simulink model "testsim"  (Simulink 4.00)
settings: Solver=ode23  StartTime=0.0  StopTime=600  MaxStep=.1  RelTol=1e-3
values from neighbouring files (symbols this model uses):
  c1 = 3    [scensim.m]
  l1 = 3    [scensim.m]
  v1 = 0.92    [scensim.m]
undefined symbols (not defined in the file or in its folder): c0, l0, p, tcap, tload, tvref, v0, x0

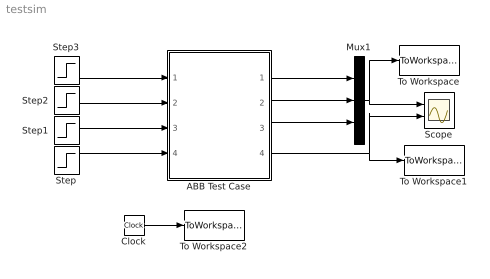
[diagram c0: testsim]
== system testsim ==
  ABB Test Case : Subsystem
  Clock : Clock
  Mux1 : Mux  Inputs=3
  Scope : Scope  NumInputPorts=2
  Step : Step  Time=100  Before=0  After=1  SampleTime=0
  Step1 : Step  Time=tvref  Before=v0  After=v1  SampleTime=0
  Step2 : Step  Time=tload  Before=l0  After=l1  SampleTime=0
  Step3 : Step  Time=tcap  Before=c0  After=c1  SampleTime=0
  To Workspace : ToWorkspace  VariableName=V  SampleTime=-1  SaveFormat=Array
  To Workspace1 : ToWorkspace  VariableName=Efd  SampleTime=-1  SaveFormat=Array
  To Workspace2 : ToWorkspace  VariableName=t  SampleTime=-1  SaveFormat=Array
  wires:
  Step2/1 -> ABB Test Case/2(LoadStep)
  Step3/1 -> ABB Test Case/1(CapStep)
  Step1/1 -> ABB Test Case/3(TapVref)
  Step/1 -> ABB Test Case/4(faulted)
  ABB Test Case/1(V2) -> Mux1/1
  ABB Test Case/2(V3) -> Mux1/2
  ABB Test Case/3(V4) -> Mux1/3
  Mux1/1 -> Scope/1, To Workspace/1
  Clock/1 -> To Workspace2/1
  ABB Test Case/4(G1Efd) -> To Workspace1/1, Scope/2

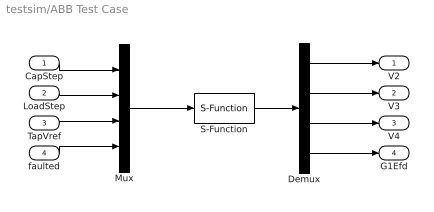
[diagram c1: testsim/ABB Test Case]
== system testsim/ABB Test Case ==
  CapStep : Inport  Port=1  LatchInput=off
  LoadStep : Inport  Port=2  LatchInput=off
  TapVref : Inport  Port=3  LatchInput=off
  faulted : Inport  Port=4  LatchInput=off
  Demux : Demux  Outputs=4  BusSelectionMode=off
  Mux : Mux  Inputs=4
  S-Function : S-Function  FunctionName=simstr  Parameters=p,x0  PortCounts=[]  SFunctionModules=''
  V2 : Outport  Port=1
  V3 : Outport  Port=2
  V4 : Outport  Port=3
  G1Efd : Outport  Port=4
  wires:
  CapStep/1 -> Mux/1
  LoadStep/1 -> Mux/2
  TapVref/1 -> Mux/3
  faulted/1 -> Mux/4
  S-Function/1 -> Demux/1
  Demux/1 -> V2/1
  Demux/2 -> V3/1
  Demux/3 -> V4/1
  Demux/4 -> G1Efd/1
  Mux/1 -> S-Function/1
